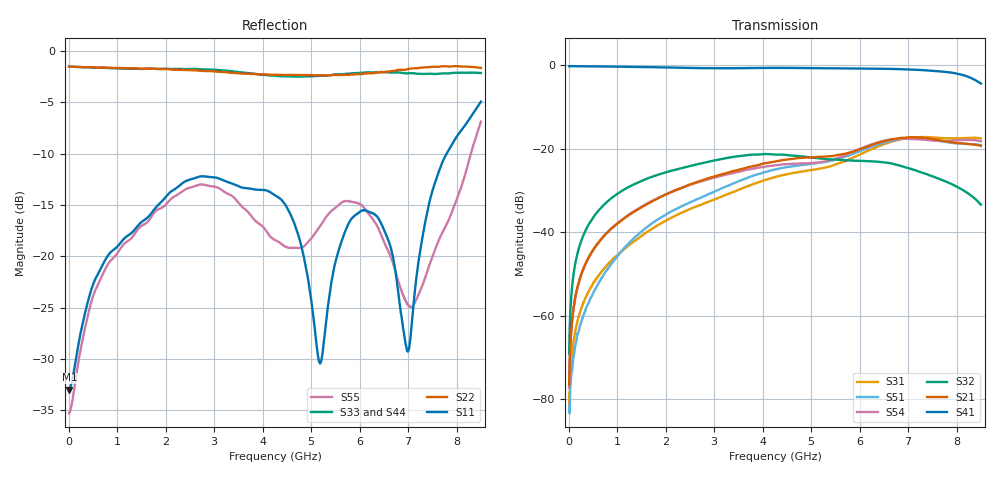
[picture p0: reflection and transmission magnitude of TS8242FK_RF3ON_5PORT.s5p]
! Created with skrf (http://scikit-rf.org).
# Hz S RI R 50.0
!freq ReS11 ImS11 ReS12 ImS12 ReS13 ImS13
! ReS14 ImS14 ReS15 ImS15
! ReS21 ImS21 ReS22 ImS22 ReS23 ImS23
! ReS24 ImS24 ReS25 ImS25
! ReS31 ImS31 ReS32 ImS32 ReS33 ImS33
! ReS34 ImS34 ReS35 ImS35
! ReS41 ImS41 ReS42 ImS42 ReS43 ImS43
! ReS44 ImS44 ReS45 ImS45
! ReS51 ImS51 ReS52 ImS52 ReS53 ImS53
! ReS54 ImS54 ReS55 ImS55
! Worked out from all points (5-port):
!   1601 points, 10 MHz to 8.5 GHz, reference 50 ohm
!   strongest paths, dB at 10 MHz, 2.132 GHz, 4.255 GHz, 6.378 GHz, 8.5 GHz:
!     S41: -0.2, -0.5, -0.6, -0.8, -4.3
!     S21: -76.5, -30.3, -23.0, -18.6, -19.3
!     S32: -69.1, -25.2, -21.4, -23.1, -33.4
!     S54: -77.3, -30.2, -24.0, -18.4, -18.2
!     S51: -81.6, -34.9, -25.0, -19.0, -19.1
!     S31: -82.8, -36.4, -26.8, -19.4, -17.5
!   lowest |S11| = -33.0 dB at 15.31 MHz (marker M1), VSWR 1.05, Z = 52.3 - j0.233 ohm
!   |S11| at or under -10 dB: start of sweep to 7.794 GHz
